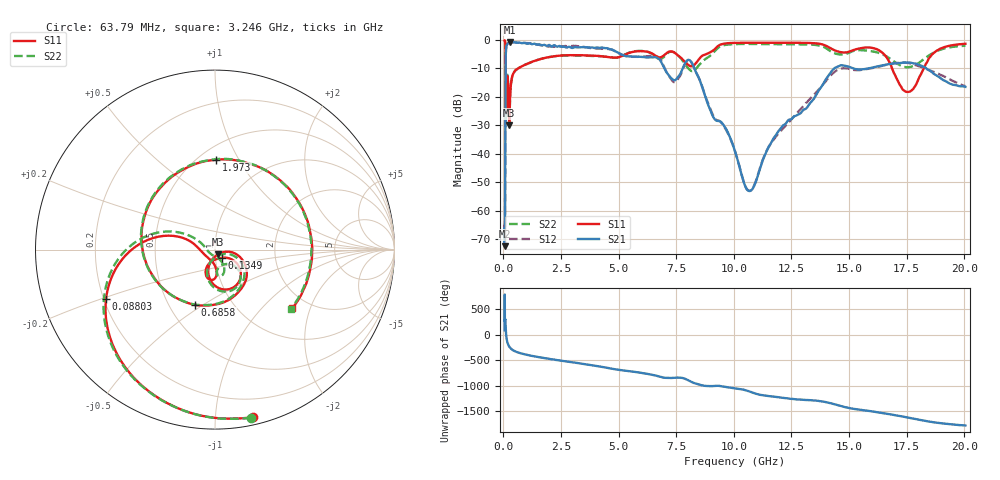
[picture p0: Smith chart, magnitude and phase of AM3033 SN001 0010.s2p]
# Hz S DB R 50
!freq MagS11 AngS11 MagS21 AngS21 MagS12 AngS12 MagS22 AngS22
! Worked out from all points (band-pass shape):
!   1601 points, 50 MHz to 20.05 GHz, reference 50 ohm
!   highest |S21| = -0.69 dB at 294.1 MHz (marker M1); lowest = -72.5 dB at 50 MHz (marker M2)
!   |S21| within 3 dB of the highest: 107.3 MHz to 4.788 GHz (4.681 GHz wide, 191 % of centre)
!   lowest |S11| = -29.9 dB at 250.4 MHz (marker M3), VSWR 1.07, Z = 51.7 - j2.78 ohm
!   |S11| at or under -10 dB: 93.56 MHz to 629.7 MHz (536.1 MHz wide, 148 % of centre); 16.87 GHz to 18.24 GHz (1.374 GHz wide, 7.82 % of centre)
!   |S22| runs from -29.5 to -0.1 dB; largest |S21 - S12| = 0.062
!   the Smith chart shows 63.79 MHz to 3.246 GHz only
!   S11 on the Smith chart (normalised r, x): 63.79 MHz: 0.06, -1.25; 88.03 MHz: 0.21, -0.21; 134.9 MHz: 1.08, -0.10; 685.8 MHz: 0.67, -0.46; 1.973 GHz: 0.60, +0.81; 3.246 GHz: 1.64, -1.52
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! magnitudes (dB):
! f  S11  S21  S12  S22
! 50 MHz  -0.2  -72.5  -66.3  -0.1
! 63.79 MHz  -0.4  -68.3  -65.3  -0.4
! 88.03 MHz  -3.5  -20.0  -20.0  -3.6
! 101.5 MHz  -23.9  -4.9  -4.9  -29.4
! 114.4 MHz  -15.4  -2.9  -2.9  -16.5
! 134.9 MHz  -24.5  -1.9  -1.9  -19.6
! 135.9 MHz  -23.7  -1.8  -1.8  -19.2
! 179.4 MHz  -12.9  -1.3  -1.3  -12.5
! 250.4 MHz  -29.9  -0.7  -0.7  -28.2
! 294.1 MHz  -18.8  -0.7  -0.7  -19.0
! 369.6 MHz  -13.1  -0.8  -0.7  -13.3
! 685.8 MHz  -9.7  -0.9  -1.0  -9.7
! 1.005 GHz  -8.5  -1.3  -1.1  -8.5
! 1.973 GHz  -6.0  -1.7  -2.3  -6.0
! 2.722 GHz  -5.4  -2.6  -2.2  -5.4
! 3.246 GHz  -5.3  -2.6  -2.1  -5.4
! 7.402 GHz  -4.3  -14.1  -14.8  -4.3
! 8.251 GHz  -9.0  -9.3  -9.4  -10.8
! 10.69 GHz  -1.0  -53.1  -53.0  -1.4
! 14.53 GHz  -4.0  -9.3  -10.4  -5.0
! 17.59 GHz  -18.2  -7.9  -8.1  -9.5
! 20.05 GHz  -1.3  -16.5  -16.2  -2.0
